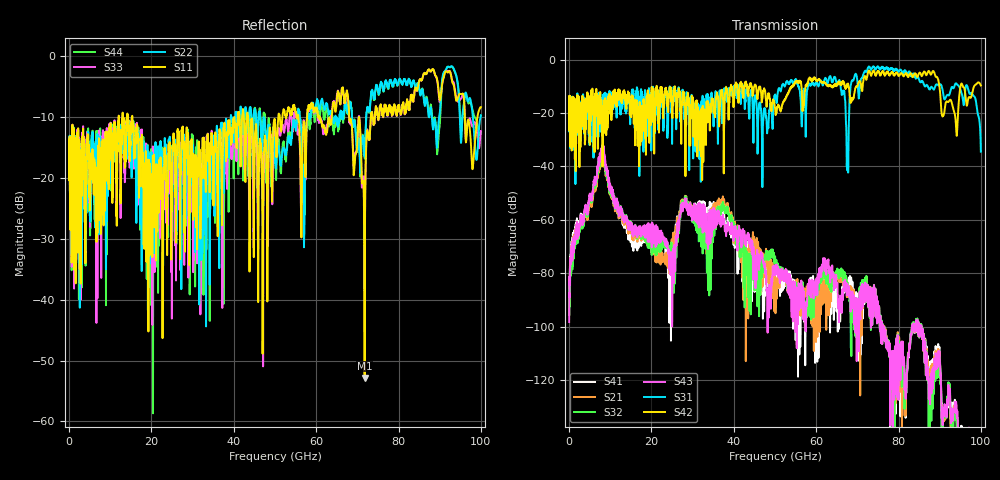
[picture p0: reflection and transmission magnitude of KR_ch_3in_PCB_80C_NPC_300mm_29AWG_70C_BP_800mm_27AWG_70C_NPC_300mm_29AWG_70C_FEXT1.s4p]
# GHz S RI R 45
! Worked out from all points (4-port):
!   4000 points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, 25 MHz to 100 GHz, reference 45 ohm
!   strongest paths, dB at 25 MHz, 25.02 GHz, 50.02 GHz, 75.03 GHz, 100 GHz:
!     S42: -20.0, -17.9, -18.0, -4.4, -9.7
!     S31: -20.0, -31.6, -13.2, -2.6, -34.5
!     S43: -98.3, -100.0, -78.4, -93.9, -155.6
!     S32: -95.2, -75.7, -73.8, -94.0, -160.2
!     S21: -89.0, -69.7, -81.4, -93.9, -161.9
!     S41: -95.8, -72.9, -81.2, -94.0, -160.9
!   lowest |S11| = -52.8 dB at 71.78 GHz (marker M1), VSWR 1.00, Z = 45.1 + j0.18 ohm
!   |S11| at or under -10 dB: start of sweep to 12.07 GHz; 15.35 GHz to 40.11 GHz (24.76 GHz wide, 89.3 % of centre); 43.48 GHz to 50.82 GHz (7.339 GHz wide, 15.6 % of centre)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
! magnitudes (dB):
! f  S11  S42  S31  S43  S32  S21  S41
! 25 MHz  -16.0  -20.0  -20.0  -98.3  -95.2  -89.0  -95.8
! 8.1 GHz  -25.2  -22.7  -20.3  -32.4  -33.8  -35.1  -33.7
! 24.35 GHz  -15.0  -13.7  -12.1  -78.7  -74.2  -75.4  -87.0
! 28.27 GHz  -15.7  -43.7  -16.1  -53.2  -52.7  -52.5  -52.9
! 67.58 GHz  -6.1  -9.6  -41.5  -84.2  -83.4  -85.4  -82.9
! 71.78 GHz  -52.8  -6.3  -4.4  -86.1  -83.0  -83.7  -86.7
! 100 GHz  -8.4  -9.7  -34.5  -155.6  -160.2  -161.9  -160.9
